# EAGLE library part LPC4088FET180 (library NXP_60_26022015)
32-bit ARM Cortex-M4 MCU; up to 512 kB flash, 96 kB SRAM; USB Device/Host/OTG; Ethernet; LCD; EMC; SPIFI The LPC408x/7x is an ARM Cortex-M4 based digital signal controller for embedded applications requiring a high level of integration and low power dissipation. The ARM Cortex-M4 is a next generation core that offers system enhancements such as low power consumption, enhanced debug features, and a high level of support block integration. The ARM Cortex-M4 CPU incorporates a 3-stage pipeline, uses a Harvard architecture with separate local instruction and data buses as well as a third bus for peripherals, and includes an internal prefetch unit that supports speculative branching. The ARM Cortex-M4 supports single-cycle digital signal processing and SIMD instructions. A hardware floating-point processor is integrated in the core for several versions of the part. The LPC408x/7x adds a specialized flash memory accelerator to accomplish optimal performance when executing code from flash. The LPC408x/7x is targeted to operate at up to 120 MHz CPU frequency. The peripheral complement of the LPC408x/7x includes up to 512 kB of flash program memory, up to 96 kB of SRAM data memory, up to 4032 byte of EEPROM data memory, External Memory controller (EMC), LCD, Ethernet, USB Device/Host/OTG, an SPI Flash Interface (SPIFI), a General Purpose DMA controller, five UARTs, three SSP controllers, three I 2 C-bus interfaces, a Quadrature Encoder Interface, four general purpose timers, two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
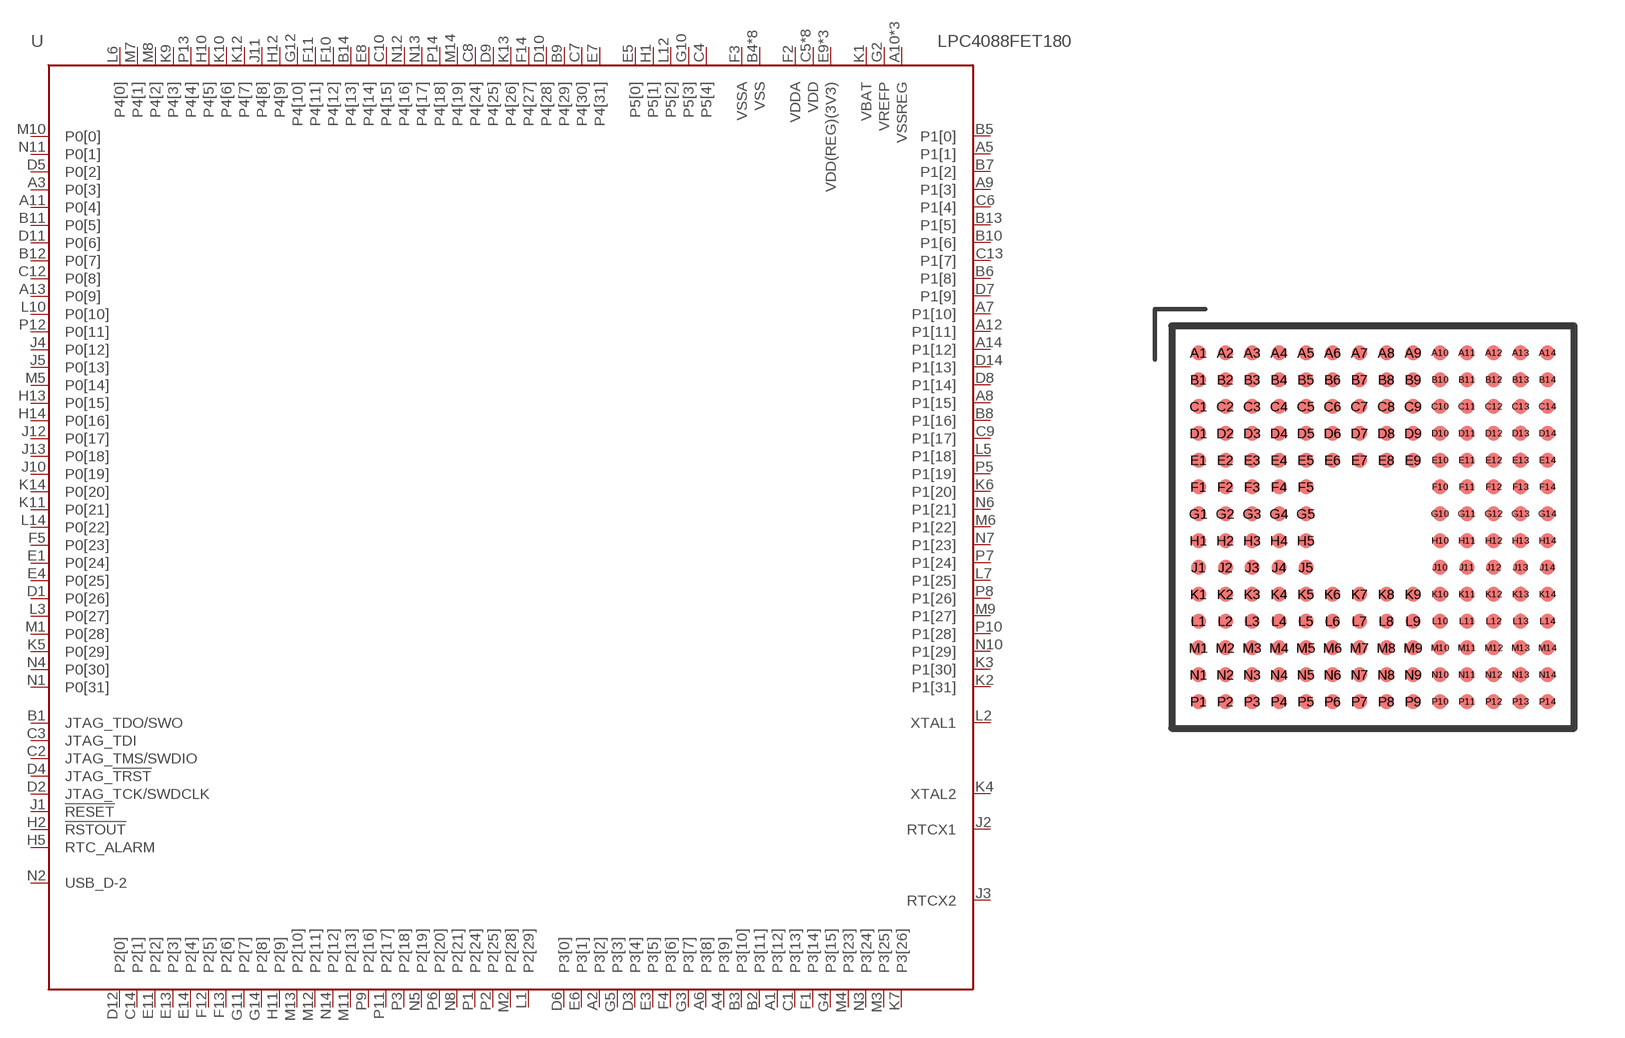
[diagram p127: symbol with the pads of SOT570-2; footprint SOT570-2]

Designator prefix U

## LPC4088FET180  [SOT570-2]
A1  P3[12]
A2  P3[2]
A3  P0[3]
A4  P3[9]
A5  P1[1]
A6  P3[8]
A7  P1[10]
A8  P1[15]
A9  P1[3]
A10  VSSREG  pwr
A11  P0[4]
A12  P1[11]
A13  P0[9]
A14  P1[12]
B1  JTAG_TDO/SWO  out
B2  P3[11]
B3  P3[10]
B4  VSS  pwr
B5  P1[0]
B6  P1[8]
B7  P1[2]
B8  P1[16]
B9  P4[29]
B10  P1[6]
B11  P0[5]
B12  P0[7]
B13  P1[5]
B14  P4[13]
C1  P3[13]
C2  JTAG_TMS/SWDIO  in
C3  JTAG_TDI  in
C4  P5[4]
C5  VDD  pwr
C6  P1[4]
C7  P4[30]
C8  P4[24]
C9  P1[17]
C10  P4[15]
C11  VSS  pwr
C12  P0[8]
C13  P1[7]
C14  P2[1]
D1  P0[26]
D2  JTAG_TCK/SWDCLK  in
D3  P3[4]
D4  JTAG_!TRST  in
D5  P0[2]
D6  P3[0]
D7  P1[9]
D8  P1[14]
D9  P4[25]
D10  P4[28]
D11  P0[6]
D12  P2[0]
D13  VSS  pwr
D14  P1[13]
E1  P0[24]
E2  VDD  pwr
E3  P3[5]
E4  P0[25]
E5  P5[0]
E6  P3[1]
E7  P4[31]
E8  P4[14]
E9  VDD(REG)(3V3)  pwr
E10  VDD  pwr
E11  P2[2]
E12  VDD  pwr
E13  P2[3]
E14  P2[4]
F1  P3[14]
F2  VDDA  pwr
F3  VSSA  pwr
F4  P3[6]
F5  P0[23]
F10  P4[12]
F11  P4[11]
F12  P2[5]
F13  P2[6]
F14  P4[27]
G1  VDD(REG)(3V3)  pwr
G2  VREFP  pwr
G3  P3[7]
G4  P3[15]
G5  P3[3]
G10  P5[3]
G11  P2[7]
G12  P4[10]
G13  VSS  pwr
G14  P2[8]
H1  P5[1]
H2  !RSTOUT!  out
H3  VSSREG  pwr
H4  VSS  pwr
H5  RTC_ALARM  out
H10  P4[5]
H11  P2[9]
H12  P4[9]
H13  P0[15]
H14  P0[16]
J1  !RESET!  in
J2  RTCX1  in
J3  RTCX2  out
J4  P0[12]
J5  P0[13]
J10  P0[19]
J11  P4[8]
J12  P0[17]
J13  P0[18]
J14  VDD  pwr
K1  VBAT  pwr
K2  P1[31]
K3  P1[30]
K4  XTAL2  out
K5  P0[29]
K6  P1[20]
K7  P3[26]
K8  VDD  pwr
K9  P4[3]
K10  P4[6]
K11  P0[21]
K12  P4[7]
K13  P4[26]
K14  P0[20]
L1  P2[29]
L2  XTAL1  in
L3  P0[27]
L4  VDD  pwr
L5  P1[18]
L6  P4[0]
L7  P1[25]
L8  VSSREG  pwr
L9  VSS  pwr
L10  P0[10]
L11  VDD  pwr
L12  P5[2]
L13  VSS  pwr
L14  P0[22]
M1  P0[28]
M2  P2[28]
M3  P3[25]
M4  P3[23]
M5  P0[14]
M6  P1[22]
M7  P4[1]
M8  P4[2]
M9  P1[27]
M10  P0[0]
M11  P2[13]
M12  P2[11]
M13  P2[10]
M14  P4[19]
N1  P0[31]
N2  USB_D-2
N3  P3[24]
N4  P0[30]
N5  P2[19]
N6  P1[21]
N7  P1[23]
N8  P2[21]
N9  VDD(REG)(3V3)  pwr
N10  P1[29]
N11  P0[1]
N12  P4[16]
N13  P4[17]
N14  P2[12]
P1  P2[24]
P2  P2[25]
P3  P2[18]
P4  VSS  pwr
P5  P1[19]
P6  P2[20]
P7  P1[24]
P8  P1[26]
P9  P2[16]
P10  P1[28]
P11  P2[17]
P12  P0[11]
P13  P4[4]
P14  P4[18]

## Footprint SOT570-2 (pad centres in mm)
SOT570-2 TFBGA180: thin fine-pitch ball grid array package; 180 balls; body 12 x 12 x 0.8 mm JEDEC: -- IEC: -- JEITA: -- Shamelessly copied from nxp_packages.lbr
smd 0.45 x 0.45: A1 -5.2,5.2; A2 -4.4,5.2; A3 -3.6,5.2; A4 -2.8,5.2; A5 -2,5.2; A6 -1.2,5.2; A7 -0.4,5.2; A8 0.4,5.2; A9 1.2,5.2; A10 2,5.2; A11 2.8,5.2; A12 3.6,5.2; A13 4.4,5.2; A14 5.2,5.2; B1 -5.2,4.4; B2 -4.4,4.4; B3 -3.6,4.4; B4 -2.8,4.4; B5 -2,4.4; B6 -1.2,4.4; B7 -0.4,4.4; B8 0.4,4.4; B9 1.2,4.4; B10 2,4.4; B11 2.8,4.4; B12 3.6,4.4; B13 4.4,4.4; B14 5.2,4.4; C1 -5.2,3.6; C2 -4.4,3.6; C3 -3.6,3.6; C4 -2.8,3.6; C5 -2,3.6; C6 -1.2,3.6; C7 -0.4,3.6; C8 0.4,3.6; C9 1.2,3.6; C10 2,3.6; C11 2.8,3.6; C12 3.6,3.6; C13 4.4,3.6; C14 5.2,3.6; D1 -5.2,2.8; D2 -4.4,2.8; D3 -3.6,2.8; D4 -2.8,2.8; D5 -2,2.8; D6 -1.2,2.8; D7 -0.4,2.8; D8 0.4,2.8; D9 1.2,2.8; D10 2,2.8; D11 2.8,2.8; D12 3.6,2.8; D13 4.4,2.8; D14 5.2,2.8; E1 -5.2,2; E2 -4.4,2; E3 -3.6,2; E4 -2.8,2; E5 -2,2; E6 -1.2,2; E7 -0.4,2; E8 0.4,2; E9 1.2,2; E10 2,2; E11 2.8,2; E12 3.6,2; E13 4.4,2; E14 5.2,2; F1 -5.2,1.2; F2 -4.4,1.2; F3 -3.6,1.2; F4 -2.8,1.2; F5 -2,1.2; F10 2,1.2; F11 2.8,1.2; F12 3.6,1.2; F13 4.4,1.2; F14 5.2,1.2; G1 -5.2,0.4; G2 -4.4,0.4; G3 -3.6,0.4; G4 -2.8,0.4; G5 -2,0.4; G10 2,0.4; G11 2.8,0.4; G12 3.6,0.4; G13 4.4,0.4; G14 5.2,0.4; H1 -5.2,-0.4; H2 -4.4,-0.4; H3 -3.6,-0.4; H4 -2.8,-0.4; H5 -2,-0.4; H10 2,-0.4; H11 2.8,-0.4; H12 3.6,-0.4; H13 4.4,-0.4; H14 5.2,-0.4; J1 -5.2,-1.2; J2 -4.4,-1.2; J3 -3.6,-1.2; J4 -2.8,-1.2; J5 -2,-1.2; J10 2,-1.2; J11 2.8,-1.2; J12 3.6,-1.2; J13 4.4,-1.2; J14 5.2,-1.2; K1 -5.2,-2; K2 -4.4,-2; K3 -3.6,-2; K4 -2.8,-2; K5 -2,-2; K6 -1.2,-2; K7 -0.4,-2; K8 0.4,-2; K9 1.2,-2; K10 2,-2; K11 2.8,-2; K12 3.6,-2; K13 4.4,-2; K14 5.2,-2; L1 -5.2,-2.8; L2 -4.4,-2.8; L3 -3.6,-2.8; L4 -2.8,-2.8; L5 -2,-2.8; L6 -1.2,-2.8; L7 -0.4,-2.8; L8 0.4,-2.8; L9 1.2,-2.8; L10 2,-2.8; L11 2.8,-2.8; L12 3.6,-2.8; L13 4.4,-2.8; L14 5.2,-2.8; M1 -5.2,-3.6; M2 -4.4,-3.6; M3 -3.6,-3.6; M4 -2.8,-3.6; M5 -2,-3.6; M6 -1.2,-3.6; M7 -0.4,-3.6; M8 0.4,-3.6; M9 1.2,-3.6; M10 2,-3.6; M11 2.8,-3.6; M12 3.6,-3.6; M13 4.4,-3.6; M14 5.2,-3.6; N1 -5.2,-4.4; N2 -4.4,-4.4; N3 -3.6,-4.4; N4 -2.8,-4.4; N5 -2,-4.4; N6 -1.2,-4.4; N7 -0.4,-4.4; N8 0.4,-4.4; N9 1.2,-4.4; N10 2,-4.4; N11 2.8,-4.4; N12 3.6,-4.4; N13 4.4,-4.4; N14 5.2,-4.4; P1 -5.2,-5.2; P2 -4.4,-5.2; P3 -3.6,-5.2; P4 -2.8,-5.2; P5 -2,-5.2; P6 -1.2,-5.2; P7 -0.4,-5.2; P8 0.4,-5.2; P9 1.2,-5.2; P10 2,-5.2; P11 2.8,-5.2; P12 3.6,-5.2; P13 4.4,-5.2; P14 5.2,-5.2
